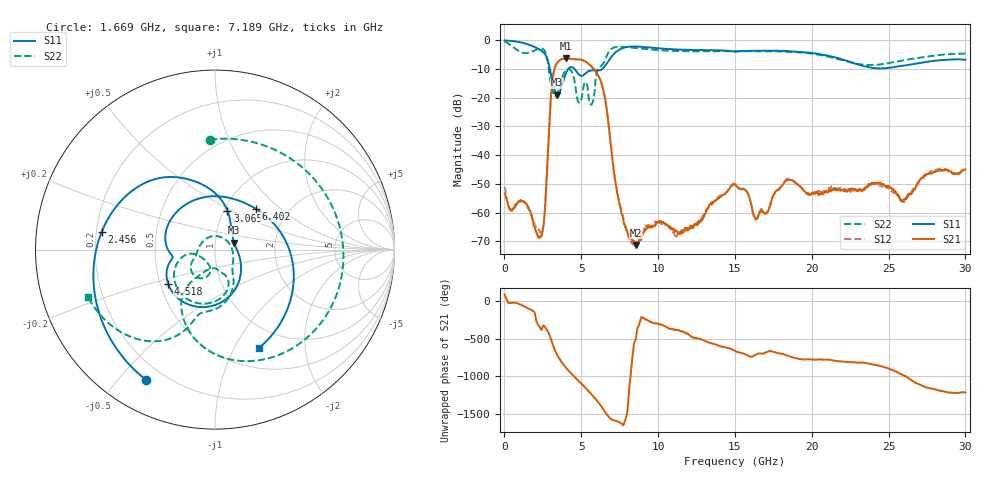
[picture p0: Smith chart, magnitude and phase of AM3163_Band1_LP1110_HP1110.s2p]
!Agilent Technologies,E8364B,MY43040894,A.07.50.67
!Agilent E8364B: A.07.50.67
!Date: Thursday, August 20, 2020 11:19:56
!Correction: S11(Full 2 Port(1,2))
!S21(Full 2 Port(1,2))
!S12(Full 2 Port(1,2))
!S22(Full 2 Port(1,2))
!S2P File: Measurements: S11, S21, S12, S22:
# Hz S  dB  R 50
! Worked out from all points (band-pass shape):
!   3201 points, 10 MHz to 30 GHz, reference 50 ohm
!   highest |S21| = -6.32 dB at 4.002 GHz (marker M1); lowest = -71.3 dB at 8.585 GHz (marker M2)
!   |S21| within 3 dB of the highest: 3.297 GHz to 5.695 GHz (2.398 GHz wide, 53.3 % of centre)
!   lowest |S11| = -19.0 dB at 3.44 GHz (marker M3), VSWR 1.25, Z = 61.6 + j4.81 ohm
!   |S11| at or under -10 dB: 2.958 GHz to 4.156 GHz (1.198 GHz wide, 33.7 % of centre); 4.557 GHz to 6.373 GHz (1.816 GHz wide, 33.2 % of centre)
!   |S22| runs from -22.4 to -0.4 dB; largest |S21 - S12| = 0.0038
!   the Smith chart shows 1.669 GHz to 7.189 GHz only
!   S11 on the Smith chart (normalised r, x): 1.669 GHz: 0.13, -0.59; 2.456 GHz: 0.22, +0.07; 3.065 GHz: 1.04, +0.48; 4.518 GHz: 0.55, -0.24; 6.402 GHz: 1.38, +0.70; 7.189 GHz: 0.73, -1.26
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1e7  -0.08 -4.7  -53.34 90.1  -50.96 -6.9  -0.38 -12.9
4.692219e8  -0.25 -32.6  -59.19 -19.9  -59.07 -14.1  -2.05 -81.4
9.378156e8  -0.61 -65.2  -56.15 -34.4  -56.38 -36.7  -3.78 -154.6
1.668822e9  -1.71 -117.8  -59.45 -107.2  -59.92 -106.5  -4.24 92.6
2.456059e9  -3.88 171.3  -67.19 1.2  -66.59 -155.5  -2.92 -38.8
3.065231e9  -12.84 72.4  -17.00 -168.8  -17.03 -168.9  -16.06 -119.8
3.440106e9  -18.99 20.1  -7.81 2.3  -7.82 2.3  -18.13 -78.5
4.002419e9  -11.54 -69.9  -6.32 -164.1  -6.34 -163.9  -10.42 -96.7
4.517872e9  -9.79 -143.4  -6.60 83.2  -6.60 83.4  -13.09 -160.9
5.014581e9  -12.43 -170.4  -6.80 -18.7  -6.79 -18.8  -20.29 -108.4
5.679984e9  -10.49 140.8  -9.24 -162.1  -9.23 -162.2  -22.27 70.1
6.401619e9  -9.86 45.2  -16.62 11.2  -16.70 11.3  -8.30 -105.1
7.188856e9  -4.43 -65.9  -48.23 -149.4  -48.24 -149.2  -2.44 -159.6
8.585266e9  -2.19 174.4  -71.30 -87.3  -70.79 125.0  -2.75 123.1
1.000979e10  -2.80 100.8  -63.33 60.5  -63.63 64.1  -3.46 65.0
1.227778e10  -3.40 10.1  -65.35 -121.5  -64.84 -32.3  -3.85 -14.6
1.5005e10  -3.97 -72.1  -50.24 58.7  -50.14 58.3  -3.81 -91.9
1.636392e10  -3.66 -104.2  -62.01 9.7  -62.42 6.0  -3.81 -125.1
2.000958e10  -4.44 163.4  -53.26 -55.2  -53.77 -49.0  -4.70 136.7
2.275554e10  -8.03 60.6  -51.69 -92.7  -52.39 -92.2  -8.00 21.0
2.500479e10  -9.65 -62.6  -50.88 -175.3  -51.57 -175.3  -7.99 -92.6
3e10  -6.82 104.6  -44.93 -135.5  -44.56 -130.3  -4.64 102.8
